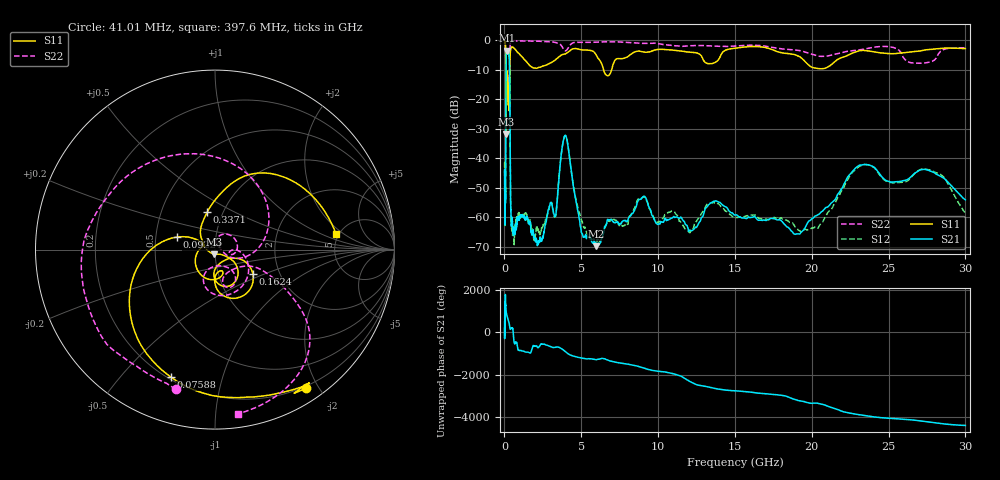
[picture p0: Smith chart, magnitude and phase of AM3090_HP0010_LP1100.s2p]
! Date/Time: Thu, Feb 28, 2019 1:55 PM
! Network Analyzer: Agilent Technologies E8364B Rev: A.07.50.67
! Sweep from 0.010 to 30.000 GHz, 1601 Points, Sweep Type: LOG
! Power Supply: 5.022 V, 0.002 A
# Hz S DB R 50
!freq MagS11 AngS11 MagS21 AngS21 MagS12 AngS12 MagS22 AngS22
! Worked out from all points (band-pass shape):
!   1601 points, 10 MHz to 30 GHz, reference 50 ohm
!   highest |S21| = -3.61 dB at 156 MHz (marker M1); lowest = -69.7 dB at 5.989 GHz (marker M2)
!   |S21| within 3 dB of the highest: 102.2 MHz to 319.9 MHz (217.6 MHz wide, 103 % of centre)
!   lowest |S11| = -31.9 dB at 99.92 MHz (marker M3), VSWR 1.05, Z = 49.5 - j2.49 ohm
!   |S11| at or under -10 dB: 90.67 MHz to 349.3 MHz (258.7 MHz wide, 118 % of centre); 6.452 GHz to 6.979 GHz (527.3 MHz wide, 7.85 % of centre)
!   |S22| runs from -32.2 to -0.1 dB; largest |S21 - S12| = 0.013
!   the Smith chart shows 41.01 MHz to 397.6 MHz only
!   S11 on the Smith chart (normalised r, x): 41.01 MHz: 0.17, -1.84; 75.88 MHz: 0.21, -0.69; 92.24 MHz: 0.65, +0.10; 162.4 MHz: 1.46, -0.42; 337.1 MHz: 0.84, +0.37; 397.6 MHz: 4.70, +1.55
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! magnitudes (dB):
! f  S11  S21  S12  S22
! 10 MHz  -0.2  -43.9  -41.4  -0.7
! 38.04 MHz  -0.5  -60.1  -59.2  -1.6
! 41.01 MHz  -0.7  -62.6  -60.2  -1.9
! 75.88 MHz  -2.5  -47.3  -47.0  -4.5
! 92.24 MHz  -13.1  -13.9  -14.0  -13.1
! 99.92 MHz  -31.9  -7.4  -7.3  -31.5
! 115.5 MHz  -13.5  -4.9  -4.8  -19.0
! 144.7 MHz  -20.3  -3.7  -3.7  -21.4
! 156 MHz  -13.8  -3.6  -3.6  -16.9
! 162.4 MHz  -12.0  -3.6  -3.6  -14.8
! 337.1 MHz  -13.5  -10.0  -10.0  -8.4
! 397.6 MHz  -3.4  -53.6  -54.1  -0.7
! 550.5 MHz  -2.5  -64.7  -65.5  -0.2
! 2.084 GHz  -9.5  -67.9  -63.4  -0.4
! 3.318 GHz  -6.7  -59.7  -59.7  -0.8
! 3.953 GHz  -4.7  -32.3  -32.2  -3.6
! 5.052 GHz  -3.3  -65.6  -61.3  -0.8
! 5.989 GHz  -5.2  -69.7  -67.5  -0.7
! 7.926 GHz  -5.9  -61.5  -62.9  -0.8
! 19.03 GHz  -5.2  -65.6  -63.5  -3.5
! 23.48 GHz  -3.5  -42.1  -42.1  -3.0
! 30 GHz  -2.9  -54.1  -58.6  -2.6
